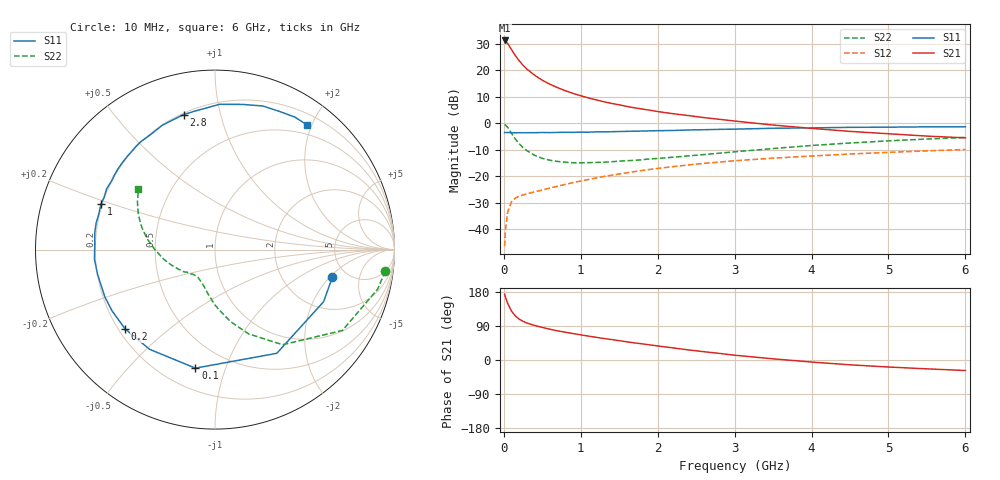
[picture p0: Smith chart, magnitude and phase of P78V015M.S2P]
! SIEMENS Small Signal Semiconductors
! BFP196
! Si NPN RF Bipolar Junction Transistor in SOT143
! VCE = 8 V  IC = 15 mA
! Common Emitter S-Parameters:  May  1996
# GHz  S  MA  R  50
!  f  S11  S21  S12  S22
! GHz  MAG  ANG  MAG  ANG  MAG  ANG  MAG  ANG
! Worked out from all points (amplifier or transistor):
!   36 points, 10 MHz to 6 GHz, reference 50 ohm
!   highest |S21| = 31.3 dB at 10 MHz (marker M1)
!   |S21| within 3 dB of that: start of sweep to 90.37 MHz
!   unconditionally stable (mu >= 1): 807.9 MHz to 3.453 GHz
!   at 250 MHz: K = 0.49, MSG = 24.5 dB, |S12| = -27.0 dB
!   at 1.4 GHz: K = 1.12, MAG = 11.5 dB, |S12| = -19.6 dB
!   at 6 GHz: K = 0.96, MSG = 2.2 dB, |S12| = -9.9 dB
!   S11 on the Smith chart (normalised r, x): 10 MHz: 3.85, -2.14; 100 MHz: 0.33, -0.79; 200 MHz: 0.23, -0.36; 1 GHz: 0.19, +0.19; 2.8 GHz: 0.21, +0.77; 6 GHz: 0.36, +1.94
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0.01  0.6719 -13.1  36.91 173.8  0.0048 84.5  0.9563 -7.2
0.02  0.671 -25.6  35.88 166.4  0.0094 76.2  0.9324 -13.7
0.05  0.6726 -59.2  32.32 149.4  0.0212 65.5  0.8406 -32.4
0.1  0.6694 -99.4  24.84 128.9  0.0331 49.2  0.6503 -54.6
0.15  0.6644 -123.3  19.04 116.0  0.0389 41.8  0.506 -68.2
0.2  0.6679 -138.6  15.26 107.8  0.0423 39.3  0.4124 -77.6
0.25  0.6674 -149.3  12.5 101.9  0.0446 37.9  0.3472 -84.7
0.3  0.6679 -156.5  10.62 97.6  0.0467 38.0  0.3063 -90.3
0.4  0.6688 -168.1  8.143 91.1  0.051 38.9  0.2498 -99.0
0.5  0.6739 -175.5  6.54 85.9  0.0552 40.8  0.2185 -105.4
0.6  0.6704 177.6  5.486 81.2  0.0603 43.1  0.2013 -110.6
0.7  0.6765 172.0  4.731 76.8  0.0652 44.6  0.1911 -115.2
0.8  0.6785 167.5  4.142 73.3  0.0705 45.5  0.1848 -119.1
1  0.684 158.2  3.328 66.4  0.0817 47.3  0.1804 -124.6
1.1  0.6833 154.5  3.034 63.0  0.0873 47.8  0.1816 -127.2
1.6  0.7078 137.0  2.09 48.0  0.117 47.1  0.1977 -139.1
2.2  0.7353 118.8  1.525 31.9  0.1528 42.8  0.23 -151.4
2.8  0.7723 103.0  1.197 17.5  0.1861 36.7  0.2738 -165.2
3.5  0.8098 88.2  0.932 3.1  0.2205 28.7  0.3351 180.0
4.5  0.8433 71.6  0.707 -12.7  0.2641 18.0  0.4267 163.0
5.5  0.8621 58.9  0.576 -23.4  0.3033 7.2  0.5076 148.4
6  0.8634 53.4  0.534 -27.7  0.3216 1.3  0.5436 141.7
